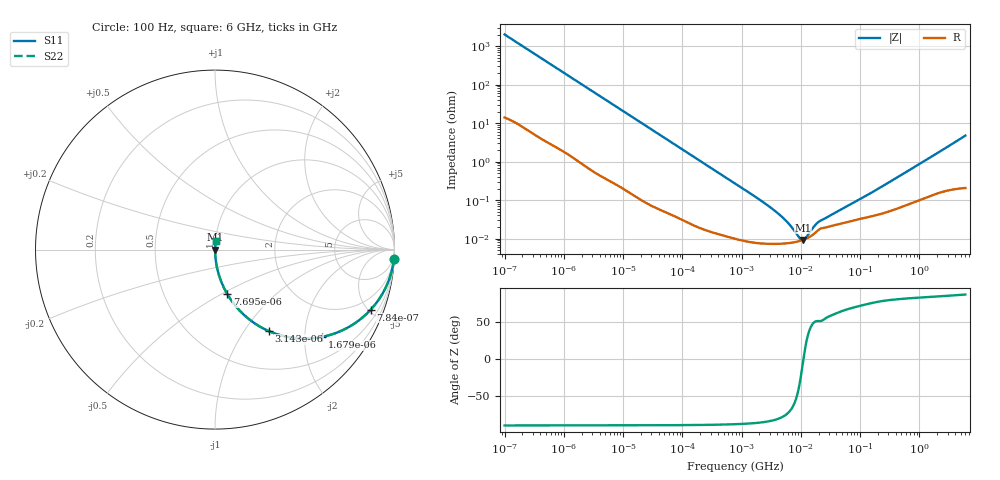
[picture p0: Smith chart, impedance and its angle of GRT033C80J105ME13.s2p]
!Murata Part Number: GRT033C80J105ME13
!These Parameters are Measured in Series Mode Connection
!Data Generated on Jun 19, 2026
!  o--ll--o
!Port1  Port2
!  o------o
!Operation Temp=25[degC], DC Bias Voltage=0[V]
!Freq. Start=100[Hz] Stop=6[GHz] 401[Steps]
# Hz S RI R 50
!Freq.(Hz) S11(Real) S11(Imag) S21(Real) S21(Imag) S12(Real) S12(Imag) S22(Real) S22(Imag)
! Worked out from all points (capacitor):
!   401 points, 100 Hz to 6 GHz, reference 50 ohm
!   read as one part in series: C = 791 nF near 109 Hz
!   lowest |Z| = 9.26 mohm at 10.87 MHz (marker M1)
!   series resonance near 11.07 MHz, so ESL is about 260 pH
!   S11 on the Smith chart (normalised r, x): 100 Hz: 1, -40; 784 Hz: 1.04, -5.18; 1.679 kHz: 1.02, -2.43; 3.143 kHz: 1.01, -1.30; 7.695 kHz: 1.01, -0.53; 6 GHz: 1.00, +0.09
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100  0.9972 -0.0497  0.00282 0.0497  0.00282 0.0497  0.9972 -0.0497
293  0.9783 -0.1417  0.0217 0.1417  0.0217 0.1417  0.9783 -0.1417
501  0.9406 -0.2323  0.0594 0.2323  0.0594 0.2323  0.9406 -0.2323
784  0.868 -0.3342  0.132 0.3342  0.132 0.3342  0.868 -0.3342
1174  0.7485 -0.4294  0.2515 0.4294  0.2515 0.4294  0.7485 -0.4294
1679  0.5953 -0.4865  0.4047 0.4865  0.4047 0.4865  0.5953 -0.4865
2008  0.5082 -0.4956  0.4918 0.4956  0.4918 0.4956  0.5082 -0.4956
3143  0.2992 -0.4537  0.7008 0.4537  0.7008 0.4537  0.2992 -0.4537
4918  0.1503 -0.353  0.8497 0.353  0.8497 0.353  0.1503 -0.353
7695  0.0686 -0.2482  0.9314 0.2482  0.9314 0.2482  0.0686 -0.2482
16473  0.0166 -0.1231  0.9834 0.1231  0.9834 0.1231  0.0166 -0.1231
40335  0.00321 -0.0512  0.9968 0.0512  0.9968 0.0512  0.00321 -0.0512
774597  0.000107 -0.00273  0.9999 0.00273  0.9999 0.00273  0.000107 -0.00273
3882480  7.32e-05 -0.000483  0.9999 0.000483  0.9999 0.000483  7.32e-05 -0.000483
6075234  7.62e-05 -0.000246  0.9999 0.000246  0.9999 0.000246  7.62e-05 -0.000246
9090158  8.49e-05 -7.61e-05  0.9999 7.61e-05  0.9999 7.61e-05  8.49e-05 -7.61e-05
1.087309e7  9.23e-05 -6.7e-06  0.9999 6.7e-06  0.9999 6.7e-06  9.23e-05 -6.7e-06
1.243624e7  0.0001 4.48e-05  0.9999 -4.48e-05  0.9999 -4.48e-05  0.0001 4.48e-05
1.555665e7  0.000123 0.000131  0.9999 -0.000131  0.9999 -0.000131  0.000123 0.000131
2.128304e7  0.00018 0.000228  0.9998 -0.000228  0.9998 -0.000228  0.00018 0.000228
3.124326e8  0.000519 0.00289  0.9995 -0.00289  0.9995 -0.00289  0.000519 0.00289
6e9  0.0043 0.0472  0.9957 -0.0472  0.9957 -0.0472  0.0043 0.0472
